(* Logix 5000 AddOnInstructionDefinition export Banner_Wireless_Site_Survey_v1_2; software revision 33.00 *)

TYPE Banner_Site_UDT :   // Data for use with Site Survey AOI.
STRUCT
   Node : INT;   // Node to gather site survey results from.
   Node_Type : INT;   // 0 = Line Powered Nodes, 1 = Battery Powered Nodes.
   Result_Green : INT;
   Result_Yellow : INT;
   Result_Red : INT;
   Result_Retry : INT;
   Control : BOOL;   // Control variable for the AOI.
END_STRUCT
END_TYPE

ADD_ON_INSTRUCTION Banner_Wireless_Site_Survey_v1_2   (* revision 1.2, vendor Banner Engineering *)
// Generate Site Survey Results for a node.  This AOI will take a small snap shot in time of the signal strength to one node.
// Revision note:
// Updated for DXM series of controllers.
VAR_IN_OUT
   Gateway_Control_Message : INT; {required}   // Commands can be sent to Gateway via this variable.
   Gateway_Input_Reserved : INT; {required}   // Compressed Site Survery results stored here.
   Gateway_Device_Message : INT; {required}   // Compressed Site Survery results stored here.
   Data : Banner_Site_UDT; {required}
END_VAR
VAR
   Lock_2 : BOOL; {access None}
   Lock_1 : BOOL; {access None}
   Timer2 : TIMER := (PRE := 60000); {access None}
   Site_Command : INT; {access None}
   TempByteSwap1 : INT; {access None}
   Lock_3 : BOOL; {access None}
   TempByteSwap2 : INT; {access None}
   Timer1 : TIMER := (PRE := 20000); {access None}
END_VAR

ROUTINE Logic   (* ladder *)
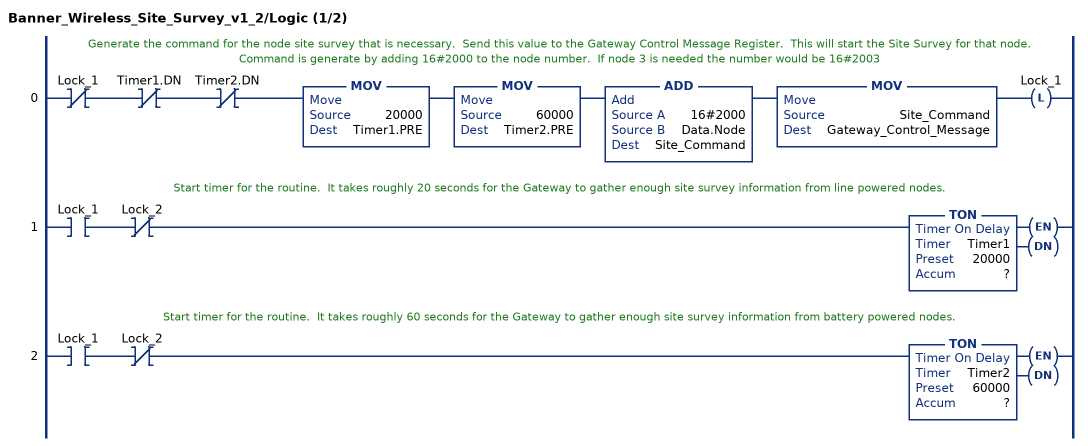
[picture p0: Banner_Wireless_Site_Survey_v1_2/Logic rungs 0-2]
   // Generate the command for the node site survey that is necessary.  Send this value to the Gateway Control Message Register.  This will start the Site Survey for that node.  Command is generate by adding 16#2000 to the node number.  If node 3 is needed the number would be 16#2003
   0: XIO(Lock_1)XIO(Timer1.DN)XIO(Timer2.DN)MOV(20000,Timer1.PRE)MOV(60000,Timer2.PRE)ADD(16#2000,Data.Node,Site_Command)MOV(Site_Command,Gateway_Control_Message)OTL(Lock_1);
   // Start timer for the routine.  It takes roughly 20 seconds for the Gateway to gather enough site survey information from line powered nodes.
   1: XIC(Lock_1)XIO(Lock_2)TON(Timer1,?,?);
   // Start timer for the routine.  It takes roughly 60 seconds for the Gateway to gather enough site survey information from battery powered nodes.
   2: XIC(Lock_1)XIO(Lock_2)TON(Timer2,?,?);
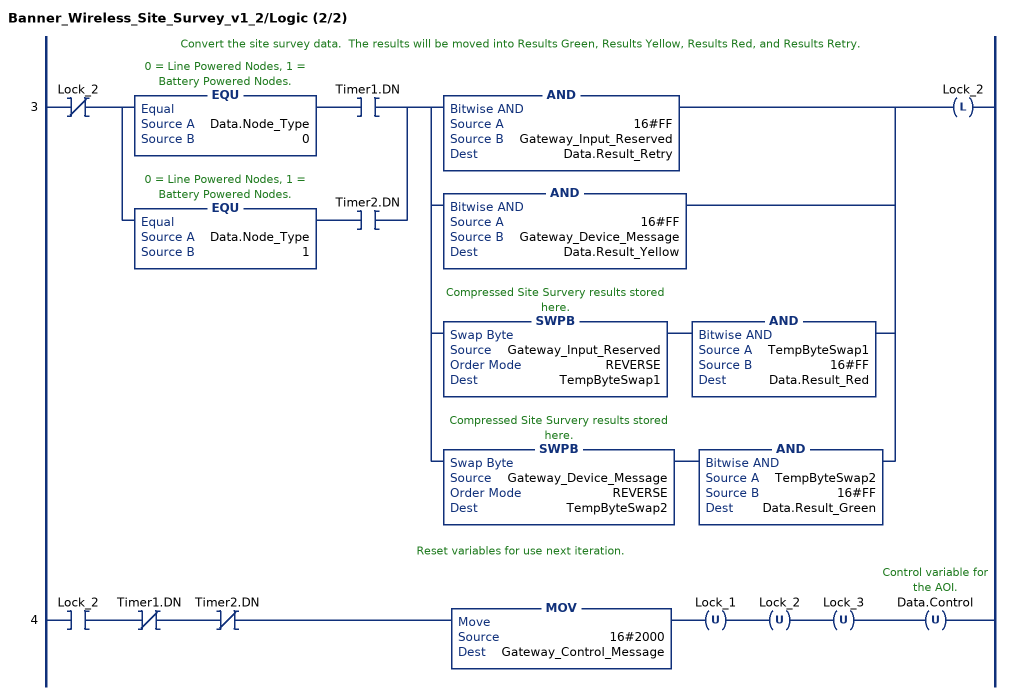
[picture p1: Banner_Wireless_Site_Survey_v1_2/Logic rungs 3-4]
   // Convert the site survey data.  The results will be moved into Results Green, Results Yellow, Results Red, and Results Retry.
   3: XIO(Lock_2)[EQU(Data.Node_Type,0) XIC(Timer1.DN) ,EQU(Data.Node_Type,1) XIC(Timer2.DN) ][AND(16#FF,Gateway_Input_Reserved,Data.Result_Retry) ,AND(16#FF,Gateway_Device_Message,Data.Result_Yellow) ,SWPB(Gateway_Input_Reserved,REVERSE,TempByteSwap1) AND(TempByteSwap1,16#FF,Data.Result_Red) ,SWPB(Gateway_Device_Message,REVERSE,TempByteSwap2) AND(TempByteSwap2,16#FF,Data.Result_Green) ]OTL(Lock_2);
   // Reset variables for use next iteration.
   4: XIC(Lock_2)XIO(Timer1.DN)XIO(Timer2.DN)MOV(16#2000,Gateway_Control_Message)OTU(Lock_1)OTU(Lock_2)OTU(Lock_3)OTU(Data.Control);
END_ROUTINE
END_ADD_ON_INSTRUCTION
